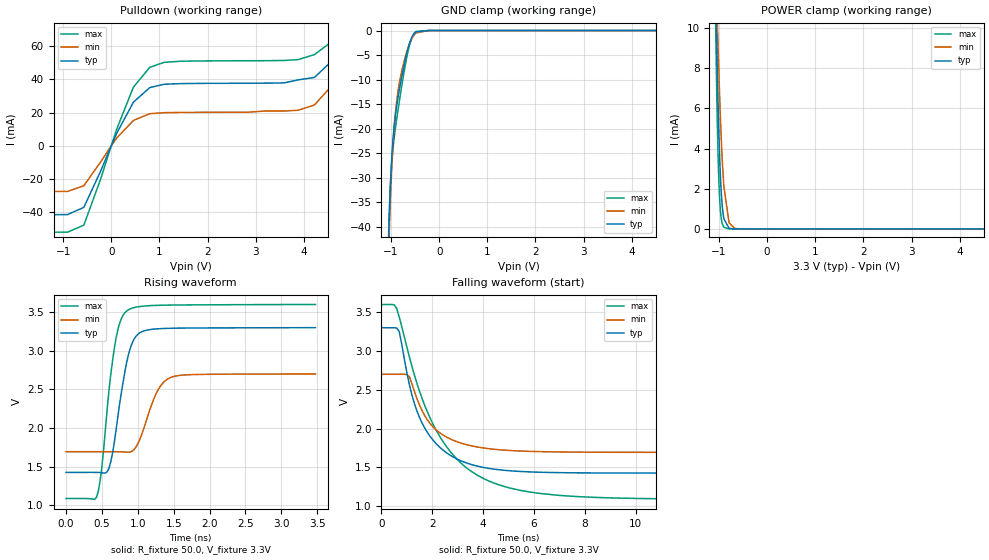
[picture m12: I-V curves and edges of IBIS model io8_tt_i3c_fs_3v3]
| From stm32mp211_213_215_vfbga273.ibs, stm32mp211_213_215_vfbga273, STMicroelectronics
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[Model]   io8_tt_i3c_fs_3v3
Model_type I/O_open_drain
Polarity   Non-Inverting
Enable   Active-Low
| CAP_THRESHOLD on pad IOTT is "UDTCAPC" :
| Rising=30.0% of vddiov33m   Falling=70.0% of vddiov33m
| C_comp min and max val. don't necessarily correlate with the min and max pvt
| but are the smallest and greatest pad capacitance found.
| var   typ   min   max
C_comp   1.30280pF  1.06453pF  2.26735pF
|C_comp_pulldown   1.30280pF  1.06453pF  2.26735pF
Vinl = 1.35V
Vinh = 1.8V
Vmeas = 1.65V   | Reference voltage for timing measurements
Cref  = 50.0pF   | Timing specification test load capacitance value
Rref  = 1.0MOhm   | Timing specification test load resistance value
Vref  = 1.815V   | Timing specification test load voltage
[Model Spec]
| TIME_THRESHOLD on pin ZIV08M is "CMOS" :
| Rising=50.0% of vddv08m   Falling=50.0% of vddv08m
Vinl 1.08570V 868.70000mV 1.21270V
Vinh 1.55630V 1.26330V 1.71030V
| variable   typ   min   max
[Temperature Range] 25.0 125.0 -40.0
| variable   typ   min   max
[Voltage Range] 3.3V 2.7V 3.6V
| variable   typ   min   max
[POWER Clamp Reference] 3.3V 2.7V 3.6V
| variable   typ   min   max
[GND Clamp Reference] 0V 0V 0V
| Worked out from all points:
|   slope of the pulldown table from 0 to 0.495 V, typ, clamps not added: 18.2 ohm
|   GND clamp passes 1 mA (typ) near -0.55 V on its own axis
|   POWER clamp passes 1 mA (typ) near -0.93 V on its own axis
|   rising waveform, R_fixture 50.0, V_fixture 3.3V: 20-80 % time 193ps typ, 240ps min, 175ps max; typ from 1.43 V to 3.3 V
|   falling waveform, R_fixture 50.0, V_fixture 3.3V: 20-80 % time 1.28ns typ, 1.26ns min, 2.05ns max; typ from 3.3 V to 1.43 V
[POWER Clamp]
-3.3V     1.353A     318.4mA    2.015A
-1.07V    12.07mA    13.62mA    10.38mA
-1.06V    10.79mA    12.67mA    8.742mA
-1.05V    9.57mA     11.75mA    7.25mA
-1.03V    7.34mA     9.996mA    4.745mA
-1V       4.587mA    7.593mA    2.212mA
-980mV    3.182mA    6.169mA    1.235mA
-950mV    1.703mA    4.334mA    479uA
-900mV    514.6uA    2.139mA    90.78uA
-790mV    28.73uA    299.8uA    2.713uA
-670mV    1.278uA    27.48uA    388.8nA
6.6V      0A         0A         0A
[GND Clamp]
-3.3V     -3.772A    -3.743A    -3.788A
-1.05V    -42.34mA   -45.44mA   -41.2mA
-1.04V    -38.9mA    -42mA      -37.88mA
-1.03V    -35.84mA   -38.88mA   -35.06mA
-1V       -28.57mA   -31.07mA   -28.88mA
-970mV    -23.48mA   -25.09mA   -24.97mA
-920mV    -18.07mA   -17.99mA   -20.63mA
-860mV    -13.91mA   -12.68mA   -16.46mA
-770mV    -9.031mA   -7.879mA   -10.78mA
-640mV    -3.394mA   -3.285mA   -3.897mA
-480mV    -254.3uA   -469.3uA   -191.8uA
6.6V      220.4nA    5.137uA    223.2nA
| variable   typ   min   max
[Pullup Reference] 3.3V 2.7V 3.6V
| variable   typ   min   max
[Pulldown Reference] 0V 0V 0V
[Pulldown]
-3.3V     -41.68mA   -27.67mA   -52.26mA
-910mV    -41.66mA   -27.66mA   -52.26mA
-570mV    -37.25mA   -24.18mA   -48.03mA
120mV     7.91mA     4.86mA     10.53mA
460mV     26.3mA     15.25mA    35.41mA
800mV     35.13mA    19.32mA    47.35mA
1.43V     37.49mA    20.09mA    50.99mA
3.88V     39.74mA    21.4mA     52mA
4.22V     41.24mA    24.57mA    55.01mA
4.56V     50.57mA    35.57mA    62.45mA
4.9V      81.48mA    69.85mA    90.32mA
6.6V      932.4mA    945.7mA    856.3mA
[Ramp]
dV/dt_r 1.12356V/192.31977ps 603.2854mV/239.18781ps 1.50665V/173.94133ps
dV/dt_f 1.12484V/1.27915ns 604.28715mV/1.25935ns 1.50794V/2.05437ns
R_load = 50.0
| Removed startup time: 0s 0s 0s  .
| Removed end time: 3.475ns.
[Rising Waveform]
R_fixture   = 50.0
V_fixture   = 3.3V
V_fixture_min = 2.7V
V_fixture_max = 3.6V
0s        1.425V     1.693V     1.087V
425ps     1.425V     1.693V     1.103V
500ps     1.421V     1.693V     1.496V
625ps     1.567V     1.693V     2.701V
725ps     2.165V     1.692V     3.281V
850ps     2.87V      1.687V     3.517V
1.025ns   3.23V      1.845V     3.571V
1.25ns    3.281V     2.433V     3.586V
1.45ns    3.29V      2.65V      3.59V
3.475ns   3.298V     2.698V     3.598V
| Removed startup time: 0s 0s 0s  .
| Removed end time: 24.9ns.
[Falling Waveform]
R_fixture   = 50.0
V_fixture   = 3.3V
V_fixture_min = 2.7V
V_fixture_max = 3.6V
0s        3.3V       2.7V       3.6V
500ps     3.3V       2.7V       3.596V
700ps     3.251V     2.7V       3.439V
1.1ns     2.566V     2.67V      2.924V
1.3ns     2.32V      2.477V     2.688V
2.1ns     1.823V     1.999V     2.012V
3.2ns     1.574V     1.805V     1.533V
4.7ns     1.466V     1.725V     1.266V
9.1ns     1.426V     1.694V     1.105V
24.9ns    1.425V     1.693V     1.087V
